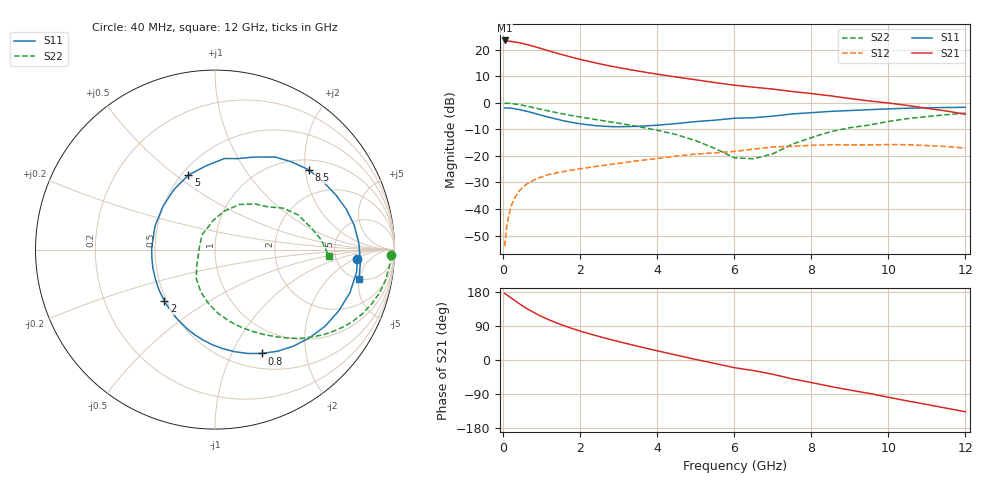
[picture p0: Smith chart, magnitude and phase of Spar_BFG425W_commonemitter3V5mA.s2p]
! Filename: 35bfg425.001
! BFG425W Field C1
! V1=8.254E-001V,V2=3.000E+000V, I1=6.088E-005A, I2=5.000E-003A
# GHz  S  MA  R 50
!  S11  S21  S12  S22
!Freq(GHz)  Mag  Ang  Mag  Ang  Mag  Ang  Mag  Ang
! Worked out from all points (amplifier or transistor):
!   44 points, 40 MHz to 12 GHz, reference 50 ohm
!   highest |S21| = 23.4 dB at 40 MHz (marker M1)
!   |S21| within 3 dB of that: start of sweep to 978.1 MHz
!   unconditionally stable (mu >= 1): 2.464 GHz to end of sweep
!   at 700 MHz: K = 0.34, MSG = 25.7 dB, |S12| = -29.9 dB
!   at 2.4 GHz: K = 0.98, MSG = 19.5 dB, |S12| = -24.0 dB
!   at 12 GHz: K = 1.50, MAG = 2.2 dB, |S12| = -17.1 dB
!   S11 on the Smith chart (normalised r, x): 40 MHz: 8.13, -2.25; 800 MHz: 0.68, -1.31; 2 GHz: 0.49, -0.33; 5 GHz: 0.54, +0.56; 8.5 GHz: 1.25, +2.09; 12 GHz: 4.95, -4.97
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0.04  0.795 -3.7  14.82 176.0  0.002 64.9  0.979 -1.9
0.1  0.799 -8.9  14.49 171.7  0.005 82.4  0.977 -5.0
0.3  0.769 -26.4  13.93 157.2  0.016 73.7  0.948 -14.8
0.5  0.72 -43.1  13.09 143.0  0.025 64.8  0.896 -23.5
0.6  0.693 -50.9  12.52 136.7  0.029 61.1  0.866 -27.4
0.8  0.635 -65.7  11.43 125.2  0.035 54.4  0.804 -34.3
1  0.579 -79.2  10.38 114.9  0.04 49.0  0.746 -40.2
1.3  0.509 -97.3  8.949 101.5  0.046 43.0  0.67 -47.6
1.6  0.452 -114.2  7.778 89.9  0.051 38.6  0.606 -53.6
2  0.402 -134.6  6.54 76.5  0.057 34.4  0.539 -60.9
2.2  0.384 -144.5  6.041 70.4  0.06 32.7  0.509 -64.3
2.6  0.361 -163.3  5.217 59.1  0.066 29.6  0.458 -71.1
3  0.353 179.0  4.573 48.6  0.072 26.5  0.411 -78.0
3.5  0.359 158.6  3.942 36.2  0.081 22.2  0.357 -87.0
4.5  0.405 124.4  3.041 12.9  0.099 11.6  0.251 -108.0
5  0.441 109.6  2.7 1.4  0.108 4.4  0.193 -122.7
6  0.51 84.2  2.137 -20.2  0.121 -9.3  0.092 -170.6
6.5  0.522 76.1  1.957 -27.9  0.134 -10.5  0.088 169.8
7.5  0.615 57.0  1.627 -49.6  0.151 -29.5  0.165 92.7
8.5  0.686 40.4  1.345 -69.9  0.162 -46.4  0.285 61.8
10.5  0.787 10.0  0.888 -108.1  0.162 -81.6  0.502 22.7
12  0.819 -11.6  0.607 -136.5  0.14 -112.5  0.637 -3.3
